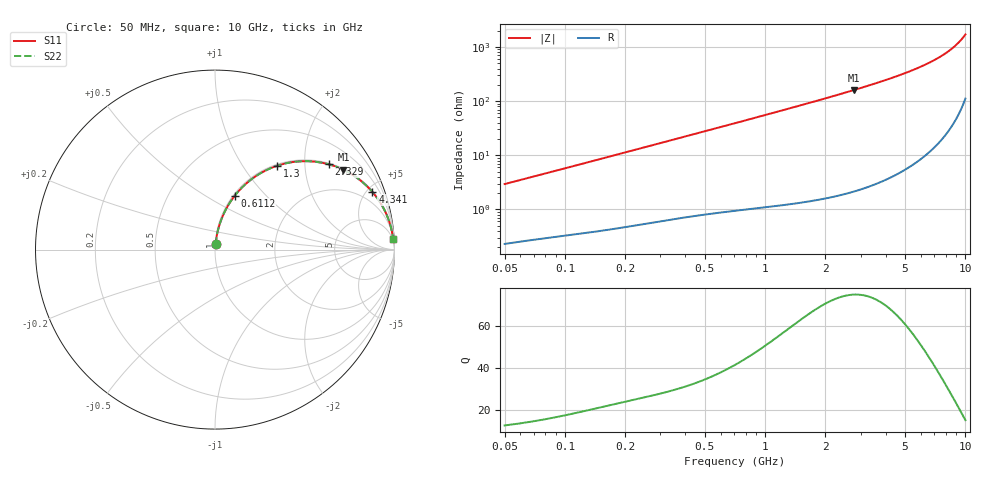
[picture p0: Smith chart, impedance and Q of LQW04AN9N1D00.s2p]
!Murata Part Number: LQW04AN9N1D00
!These Parameters are Measured in Series Mode Connection
!  o--[Z]--o
!Port1  Port2
!  o-------o
!Freq. Start=50[MHz] Stop=10[GHz], 401[Steps]
# Hz S RI R 50
!Freq.(Hz)	S 11(Real)	S 11(Imag)	S 21(Real)	S 21(Imag)	S 12(Real)	S 12(Imag)	S 22(Real)	S 22(Imag)
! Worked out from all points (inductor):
!   401 points, 50 MHz to 10 GHz, reference 50 ohm
!   read as one part in series: L = 9.25 nH near 51.34 MHz
!   highest Q = 74.8 at 2.767 GHz (marker M1), where L = 9.18 nH
!   S11 on the Smith chart (normalised r, x): 50 MHz: 1.00, +0.06; 611.2 MHz: 1.02, +0.68; 1.3 GHz: 1.02, +1.44; 2.329 GHz: 1.04, +2.65; 4.341 GHz: 1.08, +5.44; 10 GHz: 3, +34
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5e7  0.00316 0.0292  0.9968 -0.0292  0.9968 -0.0292  0.00316 0.0292
1.214486e8  0.0083 0.0684  0.9917 -0.0684  0.9917 -0.0684  0.0083 0.0684
1.930779e8  0.0162 0.1068  0.9838 -0.1068  0.9838 -0.1068  0.0162 0.1068
2.949953e8  0.032 0.159  0.968 -0.159  0.968 -0.159  0.032 0.159
4.38927e8  0.0625 0.2272  0.9375 -0.2272  0.9375 -0.2272  0.0625 0.2272
6.112328e8  0.1091 0.299  0.8909 -0.299  0.8909 -0.299  0.1091 0.299
7.071068e8  0.1387 0.3338  0.8613 -0.3338  0.8613 -0.3338  0.1387 0.3338
9.589462e8  0.2242 0.4071  0.7758 -0.4071  0.7758 -0.4071  0.2242 0.4071
1.300479e9  0.3449 0.4669  0.6551 -0.4669  0.6551 -0.4669  0.3449 0.4669
1.717543e9  0.4798 0.4922  0.5202 -0.4922  0.5202 -0.4922  0.4798 0.4922
2.329253e9  0.6347 0.4748  0.3653 -0.4748  0.3653 -0.4748  0.6347 0.4748
2.766943e9  0.7156 0.4445  0.2844 -0.4445  0.2844 -0.4445  0.7156 0.4445
3.420121e9  0.8016 0.392  0.1984 -0.392  0.1984 -0.392  0.8016 0.392
4.171863e9  0.8663 0.3331  0.1337 -0.3331  0.1337 -0.3331  0.8663 0.3331
4.34098e9  0.8773 0.3206  0.1227 -0.3206  0.1227 -0.3206  0.8773 0.3206
5.809576e9  0.9405 0.2272  0.0595 -0.2272  0.0595 -0.2272  0.9405 0.2272
6.54512e9  0.9583 0.1891  0.0417 -0.1891  0.0417 -0.1891  0.9583 0.1891
7.276762e9  0.9709 0.1556  0.0291 -0.1556  0.0291 -0.1556  0.9709 0.1556
7.983737e9  0.9795 0.1268  0.0205 -0.1268  0.0205 -0.1268  0.9795 0.1268
8.644138e9  0.9854 0.1023  0.0146 -0.1023  0.0146 -0.1023  0.9854 0.1023
9.114482e9  0.9886 0.0861  0.0114 -0.0861  0.0114 -0.0861  0.9886 0.0861
1e10  0.9928 0.058  0.00722 -0.058  0.00722 -0.058  0.9928 0.058
